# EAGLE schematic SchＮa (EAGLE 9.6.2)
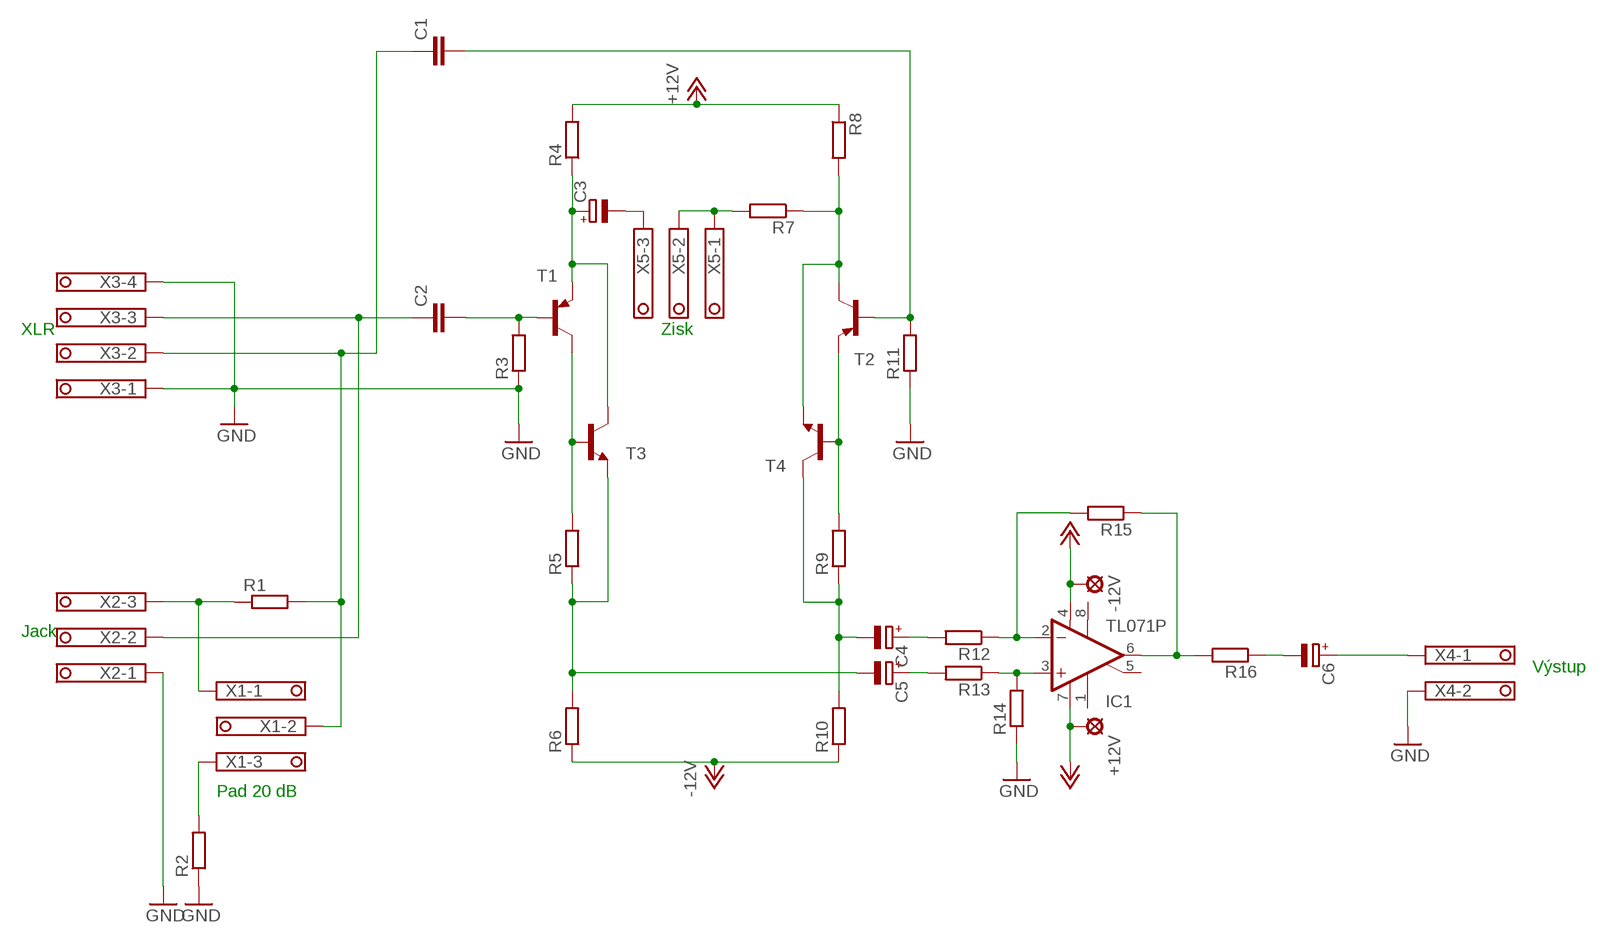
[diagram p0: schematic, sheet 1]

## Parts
+12V  LSP10  [LSP10]
-12V  LSP10  [LSP10]
C1  C-EUC1206  [C1206]
C2  C-EUC1206  [C1206]
C3  CPOL-EUE5-10.5  [E5-10,5]
C4  CPOL-EUE2-5  [E2-5]
C5  CPOL-EUE2-5  [E2-5]
C6  CPOL-EU153CLV-0605  [153CLV-0605]
IC1  TL071P  [DIL08]
R1  R-EU_M1206  [M1206]
R2  R-EU_M1206  [M1206]
R3  R-EU_M1206  [M1206]
R4  R-EU_M1206  [M1206]
R5  R-EU_M1206  [M1206]
R6  R-EU_M1206  [M1206]
R7  R-EU_M1206  [M1206]
R8  R-EU_M1206  [M1206]
R9  R-EU_M1206  [M1206]
R10  R-EU_M1206  [M1206]
R11  R-EU_M1206  [M1206]
R12  R-EU_M1206  [M1206]
R13  R-EU_M1206  [M1206]
R14  R-EU_M1206  [M1206]
R15  R-EU_M1206  [M1206]
R16  R-EU_M1206  [M1206]
T1  BC559A-PNP-TO92-EBC  [TO92-EBC]
T2  BC559A-PNP-TO92-EBC  [TO92-EBC]
T3  BC549-NPN-TO92-CBE  [TO92-CBE]
T4  BC549-NPN-TO92-CBE  [TO92-CBE]
X1  1751251  [1751251]
X2  1751251  [1751251]
X3  1751264  [1751264]
X4  1751248  [1751248]
X5  1751251  [1751251]

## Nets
+12V: +12V.MP IC1.7(V+) R4.2 R8.1
-12V: -12V.MP IC1.4(V-) R6.1 R10.1
GND: R2.1 R3.1 R11.1 R14.1 X2.1 X3.1 X3.4 X4.2
N$1: R1.1 X1.1 X2.3
N$2: C3.- X5.3
N$3: C2.1 X2.2 X3.3
N$4: R2.2 X1.3
N$5: C3.+ R4.1 T1.E T3.C
N$6: C2.2 R3.2 T1.B
N$7: R7.1 R8.2 T2.C T4.E
N$8: C1.1 R1.2 X1.2 X3.2
N$9: R7.2 X5.1 X5.2
N$10: C5.- R5.1 R6.2 T3.E
N$11: C4.- R9.1 R10.2 T4.C
N$12: R5.2 T1.C T3.B
N$13: R9.2 T2.E T4.B
N$14: C1.2 R11.2 T2.B
N$15: C4.+ R12.2
N$16: C5.+ R13.2
N$17: IC1.2(-IN) R12.1 R15.2
N$18: IC1.3(+IN) R13.1 R14.2
N$19: C6.- R16.1
N$20: IC1.6(OUT) R15.1 R16.2
N$23: C6.+ X4.1
Unconnected: IC1.1(ON1) IC1.5(ON2) IC1.8(OPT)

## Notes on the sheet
- XLR | Zisk
- Jack
- Výstup
- Pad 20 dB

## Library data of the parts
+12V -12V = solpad:LSP10: SOLDER PAD
C1 C2 = rcl:C-EU: CAPACITOR, European symbol; SPICEPREFIX: C
C3-C6 = rcl:CPOL-EU: POLARIZED CAPACITOR, European symbol; SPICEPREFIX: C
IC1 = linear:TL071: OP AMP
R1-R16 = rcl:R-EU_: RESISTOR, European symbol; SPICEPREFIX: R
T1 T2 = transistor:*-PNP-: PNP Transistror
T3 T4 = transistor:*-NPN-: NPN Transistror BF959 corrected 2008.03.06
X1 X2 X5 = con-phoenix-350:1751251: MKDS 1/ 3-3,5 Printklemme Nennstrom: 10 A Bemessungsspannung: 160 V Raster: 3,5 mm Polzahl: 3 Montageart: Löten Anschlussart: Schraubanschluss Anschlussrichtung vom Leiter zur Platine: 0° Source: http://eshop.phoenixcontact.com .. 1751251.pdf; OC_FARNELL: unknown; OC_NEWARK: unknown
X3 = con-phoenix-350:1751264: MKDS 1/ 4-3,5 Printklemme Nennstrom: 10 A Bemessungsspannung: 160 V Raster: 3,5 mm Polzahl: 4 Montageart: Löten Anschlussart: Schraubanschluss Anschlussrichtung vom Leiter zur Platine: 0° Source: http://eshop.phoenixcontact.com .. 1751264.pdf; MPN: 1751264; OC_FARNELL: unknown; OC_NEWARK: 10R0934
X4 = con-phoenix-350:1751248: MKDS 1/ 2-3,5 Printklemme; OC_FARNELL: unknown; OC_NEWARK: unknown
